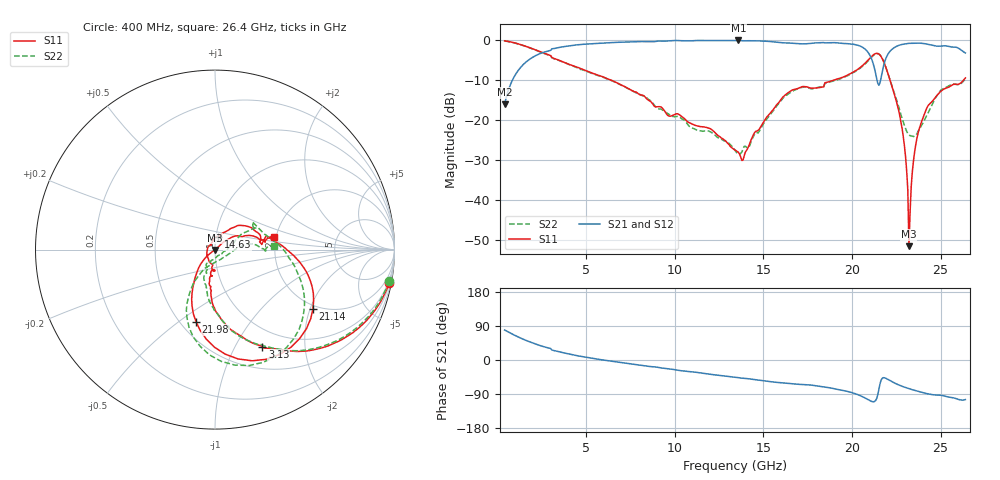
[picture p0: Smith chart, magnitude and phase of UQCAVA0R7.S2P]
!  Part Number  UQCAVA0R7  Mounting Orientation: Horizontal
!  Description: RF capacitors
!  Application: Coupling, Bypass, Tuning, DC Block
!  Filters, Matching
# GHZ S DB R 50
! Freq  |S11|  S11 Ph  |S21|  S21 Ph  |S12|  S12 Ph  |S22|  S22 Ph
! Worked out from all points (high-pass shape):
!   401 points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, 400 MHz to 26.4 GHz, reference 50 ohm
!   highest |S21| = 0.00 dB at 13.6 GHz (marker M1); lowest = -16.0 dB at 400 MHz (marker M2)
!   |S21| within 3 dB of the highest: 2.584 GHz to 20.91 GHz (18.33 GHz wide, 156 % of centre); 22.1 GHz to 26.35 GHz (4.249 GHz wide, 17.5 % of centre)
!   lowest |S11| = -51.5 dB at 23.21 GHz (marker M3), VSWR 1.01, Z = 49.8 - j0.15 ohm
!   |S11| at or under -10 dB: 6.44 GHz to 18.94 GHz (12.5 GHz wide, 98.5 % of centre); 22.15 GHz to 26.28 GHz (4.133 GHz wide, 17.1 % of centre)
!   |S22| runs from -28.5 to -0.1 dB; largest |S21 - S12| = 0.0044
!   S11 on the Smith chart (normalised r, x): 400 MHz: 1, -11; 3.13 GHz: 0.76, -1.30; 14.63 GHz: 1.03, +0.15; 21.14 GHz: 1.86, -2.10; 21.98 GHz: 0.60, -0.58; 26.4 GHz: 1.96, +0.32
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0.4  -0.10 -10.7  -16.01 79.2  -16.01 79.1  -0.14 -10.4
1.375  -1.14 -33.9  -6.39 56.4  -6.40 56.3  -1.17 -33.1
3.13  -4.41 -64.1  -2.06 25.6  -2.06 25.5  -4.48 -63.4
4.755  -7.17 -80.4  -0.99 9.1  -0.99 9.2  -7.31 -80.4
9.11  -16.59 -95.7  -0.14 -19.8  -0.13 -19.8  -17.15 -109.8
13.4  -27.49 172.5  -0.02 -45.5  -0.01 -45.5  -27.54 -79.1
13.595  -28.03 146.9  0.00 -46.6  -0.01 -46.7  -28.49 -63.4
14.635  -22.70 74.7  -0.10 -52.3  -0.09 -52.4  -23.10 -3.3
16.325  -13.31 37.7  -0.62 -61.4  -0.61 -61.5  -13.67 29.5
17.755  -11.97 10.0  -0.69 -66.5  -0.68 -66.7  -12.11 30.5
20.225  -7.56 -2.2  -1.09 -89.5  -1.08 -89.7  -7.70 -5.9
21.135  -3.89 -31.4  -4.97 -109.7  -4.96 -109.8  -4.08 -39.0
21.525  -3.42 -65.0  -11.23 -75.8  -11.21 -75.9  -3.43 -73.5
21.98  -7.63 -104.7  -3.85 -50.0  -3.84 -50.2  -7.68 -112.1
22.11  -9.40 -112.2  -2.92 -53.6  -2.91 -53.8  -9.44 -117.5
22.825  -21.94 -138.2  -1.00 -69.3  -0.99 -69.5  -19.49 -114.6
23.215  -51.55 -145.3  -0.72 -75.7  -0.71 -75.9  -23.60 -79.5
23.345  -36.46 38.4  -0.71 -77.6  -0.70 -77.8  -23.91 -65.5
23.67  -24.38 41.5  -0.68 -81.6  -0.67 -81.8  -23.36 -31.2
24.19  -17.26 33.5  -0.88 -88.4  -0.87 -88.6  -19.04 -0.2
25.035  -12.66 18.2  -1.39 -93.2  -1.38 -93.4  -12.38 4.8
26.4  -9.39 12.4  -3.14 -104.5  -3.13 -104.7  -9.62 3.8
